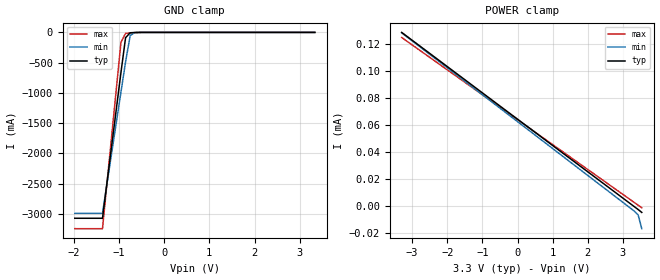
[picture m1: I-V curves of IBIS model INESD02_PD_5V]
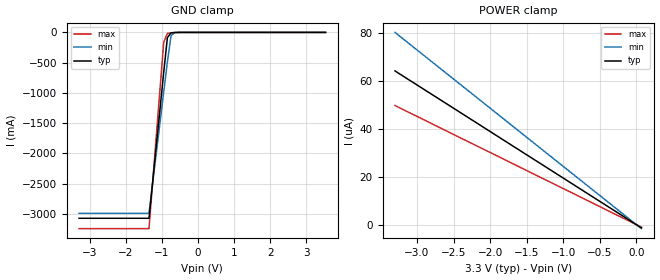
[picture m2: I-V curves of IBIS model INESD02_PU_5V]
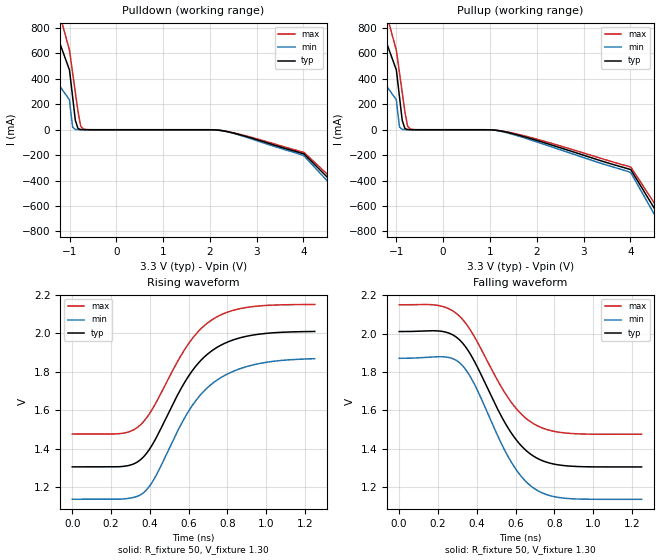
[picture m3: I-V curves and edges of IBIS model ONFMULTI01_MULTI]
|   This file is an IBIS representation of the   |
|   Integrated Device Technology, Inc.   |
|   ICS813252I-02   |
|   VCXO JITTER ATTENUATOR/MULTIPLIER FEMTOCLOCK MULTIPLIER   |
[IBIS Ver]   4.1
[File name]   813252i_02_3v3.ibs
[File Rev]   1.2
|Revision History
|Rev 1.0 Nov 05, 2008 IBIS
|Rev 1.1 Jan 19th, 2010
|Updated the model to 1000 points on rise/fall waveforms.
|Rev 1.2 Corrected the INESD02_PD_5V Voltage range to typ +/- 5%.
|Removed ground clamp data from the Power clamp I-V curves.
|Added Temperature range keyword. Temperature Range reflects the
|temperatures used in the SPICE simulations.
|Updated C_comp values for each model.  The values were obtained
|from simulation using an LC Tank circuit.
[Notes] This model complies to IBIS Quality standard IQ3S.  IBIS simulation results
have been correlated to the SPICE waveforms.
It should be noted that currents have been limited to 3A or less in the
Clamp and Pullup/Pulldown I-V curves because a breakdown in the CMOS modelling
predicts extreme currents.  This is beyond the device ratings and in a real system
would lead to catastrophic failure.
[Date]   29  March 2010
[Source]   Originated at Integrated Device Technology, Inc.
[Disclaimer]
IDT hereby grants the user of this IBIS model a non-exclusive,
nontransferable license to use this IBIS model under the following terms.
Before using this IBIS model, the user should read this license.
If the user does not accept these terms,  the IBIS model should be
returned to IDT within 30 days.
   The user is granted this license only to use the IBIS model and
is not granted rights to sell, load, rent, lease or license the IBIS
model in whole or in part, or in modified form to anyone other than
user. User may modify the IBIS model to suit its specific
applications but rights to derivative works and such modifications
shall belong to IDT.
   This IBIS model is provided on an "AS IS" basis and IDT makes
absolutely no warranty with respect to the information contained
herein. IDT DISCLAIMS AND CUSTOMER WAIVES ALL WARRANTIES, EXPRESS
OR IMPLIED, INCLUDING WARRANTIES OF MERCHANTABILITY OR FITNESS FOR
A PARTICULAR PURPOSE. The entire risk as to quality and performance
is with the Customer. ACCORDINGLY, IN NO EVENT SHALL THE COMPANY BE
LIABLE FOR ANY DAMAGES, WHETHER IN CONTRACT OR TORT,INCLUDING ANY
LOST PROFITS OR OTHER INCIDENTAL, CONSEQUENTIAL, EXEMPLARY, OR
PUNITIVE DAMAGES ARISING OUT OF THE USE OR APPLICATION OF THE IBIS
model provided in this package. Further, IDT reserves the right to
make changes without notice to any product herein to improve
reliability, function, or design. IDT does not convey any license
under patent rights or any other intellectual property rights,
including those of third parties.
   IDT is not obligated to provide maintenance or support
for the licensed IBIS model.
[Copyright]   Copyright 2008 by Integrated Device Technology, Inc.
[Component]   ICS813252CKI-03
[Manufacturer] Integrated Device Technology, Inc.
[Package]
|QFN 32
|lead + wire   typ   min   max
R_pkg   72.4655m   58.886m   86.045m
L_pkg   1.47175nH   1.11650nH   1.77850nH
C_pkg   0.07747pF   0.07444pF   0.08050pF
[Pin] signal_name   model_name   R_pin   L_pin   C_pin
1   LF1   NC   86.045m   1.77850nH   0.08050pF
2   LF0   NC   76.996m   1.55783nH   0.07848pF
3   ISET   NC   67.941m   1.33717nH   0.07646pF
4   VEE   GND   58.886m   1.11650nH   0.07444pF
5   CLK_SEL   INESD02_PD_5V   58.886m   1.11650nH   0.07444pF
6   VCC   POWER   67.941m   1.33717nH   0.07646pF
7   RESERVED   NC   76.996m   1.55783nH   0.07848pF
8   VEE   GND   86.045m   1.77850nH   0.08050pF
9   PDSEL_2   INESD02_PU_5V   86.045m   1.77850nH   0.08050pF
10   PDSEL_1   INESD02_PU_5V   76.996m   1.55783nH   0.07848pF
11   PDSEL_0   INESD02_PU_5V   67.941m   1.33717nH   0.07646pF
12   VCC   POWER   58.886m   1.11650nH   0.07444pF
13   VCCA   POWER   58.886m   1.11650nH   0.07444pF
14   ODBSEL_1   INESD02_PD_5V   67.941m   1.33717nH   0.07646pF
15   ODBSEL_0   INESD02_PD_5V   76.996m   1.55783nH   0.07848pF
16   ODASEL_1   INESD02_PD_5V   86.045m   1.77850nH   0.08050pF
17   ODASEL_0   INESD02_PD_5V   86.045m   1.77850nH   0.08050pF
18   VEE   GND   76.996m   1.55783nH   0.07848pF
19   QA   ONFMULTI01_MULTI   67.941m   1.33717nH   0.07646pF
20   nQA   ONFMULTI01_MULTI   58.886m   1.11650nH   0.07444pF
21   VCCO   POWER   58.886m   1.11650nH   0.07444pF
22   QB   ONFMULTI01_MULTI   67.941m   1.33717nH   0.07646pF
23   nQB   ONFMULTI01_MULTI   76.996m   1.55783nH   0.07848pF
24   VEE   GND   86.045m   1.77850nH   0.08050pF
25   nCLK1   INESD02_PMID_5V   86.045m   1.77850nH   0.08050pF
26   CLK1   INESD02_PD_5V   76.996m   1.55783nH   0.07848pF
27   VCC   POWER   67.941m   1.33717nH   0.07646pF
28   nCLK0   INESD02_PMID_5V   58.886m   1.11650nH   0.07444pF
29   CLK0   INESD02_PD_5V   58.886m   1.11650nH   0.07444pF
30   XTAL_OUT   NC   67.941m   1.33717nH   0.07646pF
31   XTAL_IN   NC   76.996m   1.55783nH   0.07848pF
32   VCCX   POWER   86.045m   1.77850nH   0.08050pF
[Diff Pin]  inv_pin  vdiff tdelay_typ tdelay_min  tdelay_max
|Input
26   25   0.15  0   0   0
29   28   0.15  0   0   0
|Output
19   20   NA   0   0   0
22   23   NA   0   0   0
| Models and submodels in the file (4): INESD02_PD_5V (Input), INESD02_PU_5V (Input), ONFMULTI01_MULTI (Output_ECL), INESD02_PMID_5V (Input)
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[Model]   INESD02_PD_5V
Model_type  Input
Polarity   Non-Inverting
Vinl = 0.8V
Vinh = 2.0V
|   typ   min   max
C_comp   2.21pF   2.11pF   2.32pF
|   typ   min   max
[Temperature Range] 25   -40   85
[Voltage range]  3.3V   3.135V   3.465V
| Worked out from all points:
|   GND clamp passes 1 mA (typ) near -0.58 V on its own axis
[GND_clamp]
|Voltage   I(typ)   I(min)   I(max)
-1.973V   -3.072A    -2.991A    -3.244A
-1.361V   -3.072A    -2.991A    -3.244A
-952.6mV  -663.4mA   -987.4mA   -164.5mA
-850.5mV  -87.6mA    -487.5mA   -16.04mA
-748.5mV  -6.317mA   -52.72mA   -9.171mA
-646.4mV  -1.91mA    -2.66mA    -4.148mA
3.334V    64.95uA    66.45uA    61.52uA
[POWER_clamp]
|Voltage   I(typ)   I(min)   I(max)
-3.3V     128.6uA    128.3uA    124.8uA
3.334V    -662.9nA   -4.004uA   2.417uA
3.436V    -2.655uA   -6.645uA   533.6nA
3.538V    -4.767uA   -16.82uA   -1.35uA
[Model]   INESD02_PU_5V
Model_type   Input
Polarity   Non-Inverting
Vinl = 0.8V
Vinh = 2.0V
|   typ   min   max
C_comp   2.21pF   2.11pF   2.32pF
|   typ   min   max
[Temperature Range] 25   -40   85
[Voltage range]  3.3V   3.135V   3.465V
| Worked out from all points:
|   GND clamp passes 1 mA (typ) near -0.58 V on its own axis
[GND_clamp]
|Voltage   I(typ)   I(min)   I(max)
-3.3V     -3.072A    -2.991A    -3.244A
-1.361V   -3.072A    -2.991A    -3.244A
-952.6mV  -663.5mA   -987.5mA   -164.6mA
-850.5mV  -87.67mA   -487.6mA   -16.09mA
-748.5mV  -6.381mA   -52.8mA    -9.221mA
-646.4mV  -1.974mA   -2.739mA   -4.198mA
3.538V    4.64uA     9.821uA    1.104uA
[POWER_clamp]
|Voltage   I(typ)   I(min)   I(max)
-3.3V     64.29uA    80.4uA     49.82uA
-2.484V   48.38uA    60.5uA     37.49uA
-1.973V   38.44uA    48.07uA    29.79uA
68.04mV   -1.325uA   -1.657uA   -1.027uA
[Model]   ONFMULTI01_MULTI
Model_type   Output_ECL
Polarity   Non-Inverting
|   typ   min   max
C_comp   1.59pF   1.49pF   1.61pF
Vmeas = 1.61V
Rref = 50
Cref = 0
[Model Spec]
Vref 1.3V   1.135V  1.465V
|   typ   min   max
[Temperature Range]   25   -40   85
[Voltage range]   3.3V   3.135V   3.465V
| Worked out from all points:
|   rising waveform, R_fixture 50, V_fixture 1.30: 20-80 % time 245ps typ, 258ps min, 239ps max; typ from 1.3 V to 2.01 V
|   falling waveform, R_fixture 50, V_fixture 1.30: 20-80 % time 223ps typ, 214ps min, 233ps max; typ from 2.01 V to 1.3 V
[Pulldown]
|Voltage   I (typ)   I (min)   I (max)
-3.3V     2.816A     1.413A     3.741A
-2.38V    1.877A     942.1mA    2.494A
-1.46V    938.6mA    471.1mA    1.247A
-1V       469.3mA    235.5mA    623.5mA
-932.6mV  255.1mA    20.47mA    444.9mA
-875.3mV  73.65mA    2.306mA    293mA
-760.6mV  1.771mA    208.5uA    27.6mA
-703.2mV  533.9uA    59.86uA    5.212mA
2.566V    -32mA      -34.86mA   -29.75mA
4.01V     -190.1mA   -205.1mA   -178.3mA
5.564V    -760.4mA   -820.3mA   -713mA
6.6V      -1.141A    -1.23A     -1.07A
[Pullup]
|Voltage   I (typ)   I (min)   I (max)
-3.3V     2.816A     1.413A     3.741A
-2.38V    1.877A     942.1mA    2.494A
-1.46V    938.6mA    471.1mA    1.247A
-1V       469.3mA    235.5mA    623.5mA
-932.6mV  255.1mA    20.47mA    444.9mA
-875.3mV  73.65mA    2.306mA    293mA
-703.2mV  533.9uA    59.86uA    5.212mA
1.19V     -7.513mA   -8.763mA   -6.469mA
4.01V     -313.9mA   -337.8mA   -293.3mA
4.528V    -627.9mA   -675.6mA   -586.6mA
5.046V    -941.8mA   -1.013A    -879.9mA
6.6V      -1.884A    -2.027A    -1.76A
[Ramp]
|   typ   min   max
dV/dt_r   0.564/0.385n   0.585/0.411n   0.54/0.37n
dV/dt_f   0.567/0.339n   0.594/0.324n   0.541/0.355n
R_load =   50.0000
[Rising Waveform]
R_fixture = 50
V_fixture = 1.30   | VCC_typ - 2V
V_fixture_max = 1.465   | VCC_max - 2V
V_fixture_min = 1.135   | VCC_min - 2V
C_fixture = 0.0p
| Time   typ   min   max
0s        1.305V     1.136V     1.475V
264ps     1.307V     1.138V     1.48V
319.1ps   1.321V     1.146V     1.499V
366.6ps   1.356V     1.169V     1.539V
427.9ps   1.447V     1.252V     1.632V
600.6ps   1.779V     1.596V     1.948V
669.4ps   1.866V     1.689V     2.03V
747ps     1.927V     1.757V     2.086V
947.2ps   1.993V     1.839V     2.141V
1.25ns    2.01V      1.868V     2.15V
[Falling Waveform]
R_fixture = 50
V_fixture = 1.30   | VCC_typ - 2V
V_fixture_max = 1.465   | VCC_max - 2V
V_fixture_min = 1.135   | VCC_min - 2V
C_fixture = 0.0p
| Time   typ   min   max
0s        2.011V     1.871V     2.15V
209ps     2.013V     1.88V      2.145V
317.8ps   1.961V     1.842V     2.084V
386.6ps   1.858V     1.739V     1.986V
514.3ps   1.593V     1.454V     1.744V
578.1ps   1.482V     1.33V      1.642V
643.1ps   1.401V     1.24V      1.568V
712ps     1.35V      1.183V     1.52V
865.9ps   1.31V      1.141V     1.481V
1.25ns    1.305V     1.136V     1.476V
